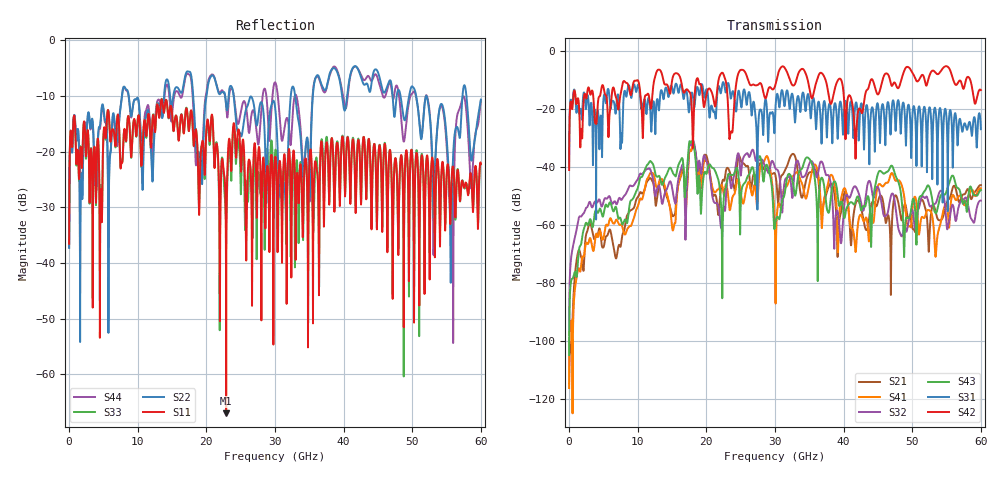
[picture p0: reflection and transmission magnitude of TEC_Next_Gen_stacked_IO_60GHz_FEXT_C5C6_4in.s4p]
!! CHANNEL DESCRIPTION:  Next Generation 28Gbps Press-fit Stacked I/O Connector
!!  with 4" 5-6-5 Megtron 6 Stripline trace on host side and 1.25" 7-5-7 Megtron 6 Microstrip trace on plug side
!! HOST PCB DESCRIPTION:  PCB thickness 3.425 mm
!!  26 Layer Board, 15 GND planes, 4 Layer route-out on Layers 7,11,17,21, 8mil stub on vias
!!  Pairs on following layers
!!  Layer 07 - A02A03 A14A15 D05D06
!!  Layer 11 - D020D3 C05C06 D14D15
!!  Layer 17 - C02C03 B05B06 C14C15
!!  Layer 21 - B02B03 A05A06 B14B15
!! CONNECTOR DESCRIPTION:  Next Generation 28Gbps Press-fit Stacked I/O Connector
!! PLUG-IN CARD DESCRIPTION:  PCB thickness 1mm thick
!!  6 Layer Board, 4 GND planes, 0.35 x 1.4mm mating pads
!!  Micro-strip diff traces referenced to GND plane 3mils down, 2nd GND plane 17mils from top of board
!!  PCB GND planes are symmetric
!! MODEL DESCRIPTION: TE Connectivity S-parameter model produced from Macro-model, Extracted .s4p FEXT (Victim B05B06 - Aggressor C05C06)
!! MODEL DATE: 5/15/2014 CR32f, FPR23
!! MODEL STATUS: Developmental
!! MODEL GEOMETRY: 4 Rows - Rows A, B, C, D. 3 pairs in each row, 12 total pairs
!! MODEL FREQUENCY RANGE: DC to 60 GHz in 10 MHz frequency steps
!! MODEL EDGE RATE LIMITATION: 8.33 ps (Using conservative 0.5/Fmax rule of thumb)
!! TIME-DOMAIN TRANSFORM CAUTIONS:
!! 1.) Do not simulate transient edge rates faster than the number listed above.  Edge
!!  rates faster than this number contain significant spectral content at frequencies
!!  above the model's highest frequency.
!! 2.) Even when simulating edge rates that are slower than the number listed above, be
!!  aware that the best time resolution possible with a direct iFFT is (1 / 2Fmax).
!!  As a result, time resolution is typically not adequate for most time-domain
!!  simulations unless tricks such as frequency-domain zero-padding and windowing are
!!  used to minimize leakage and aliasing.
!! 3.) Because the model has a uniform frequency step, a direct iFFT will result in an
!!  impulse that that has a time length given by either (1 / Fstep) or (1 / 2Fstep),
!!  depending on the transform being used.  Care has been taken in selecting the
!!  frequency step to ensure a settled impulse response for the model.  Therefore,
!!  convolution with the model's impulse response should present no issues.  However,
!!  if directly concatenating s-parameter models in the frequency domain a user must
!!  either interpolate necessary interim frequencies or complete impulse response
!!  zero-padding.  Impulse response zero-padding is more difficult, but more accurate.
!! PORT DEFINITIONS:
!! Port  1  ----->  Host C05		B05 Module <-----  Port  2
!! Port  3  ----->  Host C06		B06 Module <-----  Port  4
! Touchstone data
! Created: 29-Sep-2014 by IdEM R2011 (7.0.3)
# Hz S MA R 50
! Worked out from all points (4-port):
!   6000 points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, 10 MHz to 60 GHz, reference 50 ohm
!   strongest paths, dB at 10 MHz, 15.01 GHz, 30.01 GHz, 45.01 GHz, 60 GHz:
!     S42: -41.0, -10.1, -12.0, -14.9, -13.4
!     S31: -40.1, -12.4, -23.0, -18.4, -26.9
!     S43: -104.9, -41.3, -60.0, -42.2, -47.9
!     S32: -98.0, -47.0, -40.2, -46.9, -51.6
!     S41: -116.3, -60.7, -63.5, -46.4, -47.3
!     S21: -114.6, -56.6, -42.4, -51.9, -46.2
!   lowest |S11| = -67.0 dB at 22.89 GHz (marker M1), VSWR 1.00, Z = 50 + j0.0436 ohm
!   |S11| at or under -10 dB: start of sweep to end of sweep
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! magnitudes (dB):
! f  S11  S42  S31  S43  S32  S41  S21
! 10 MHz  -36.6  -41.0  -40.1  -104.9  -98.0  -116.3  -114.6
! 11.72 GHz  -14.6  -16.7  -17.2  -38.1  -40.4  -42.5  -43.9
! 22.89 GHz  -67.0  -11.0  -13.8  -46.1  -49.2  -46.0  -40.9
! 41.76 GHz  -31.0  -36.1  -17.9  -51.7  -46.8  -69.3  -52.5
! 50.09 GHz  -23.5  -7.6  -20.3  -51.0  -55.4  -53.1  -61.4
! 55.58 GHz  -32.1  -6.9  -20.4  -44.1  -55.8  -53.3  -50.1
! 60 GHz  -22.2  -13.4  -26.9  -47.9  -51.6  -47.3  -46.2
